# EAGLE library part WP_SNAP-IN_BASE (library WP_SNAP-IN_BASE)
SIERRA WIRELESS - WP SNAP-IN BASE - SNAP-IN SOCKET BASE FOR WP SERIES MCU Source: Datasheet
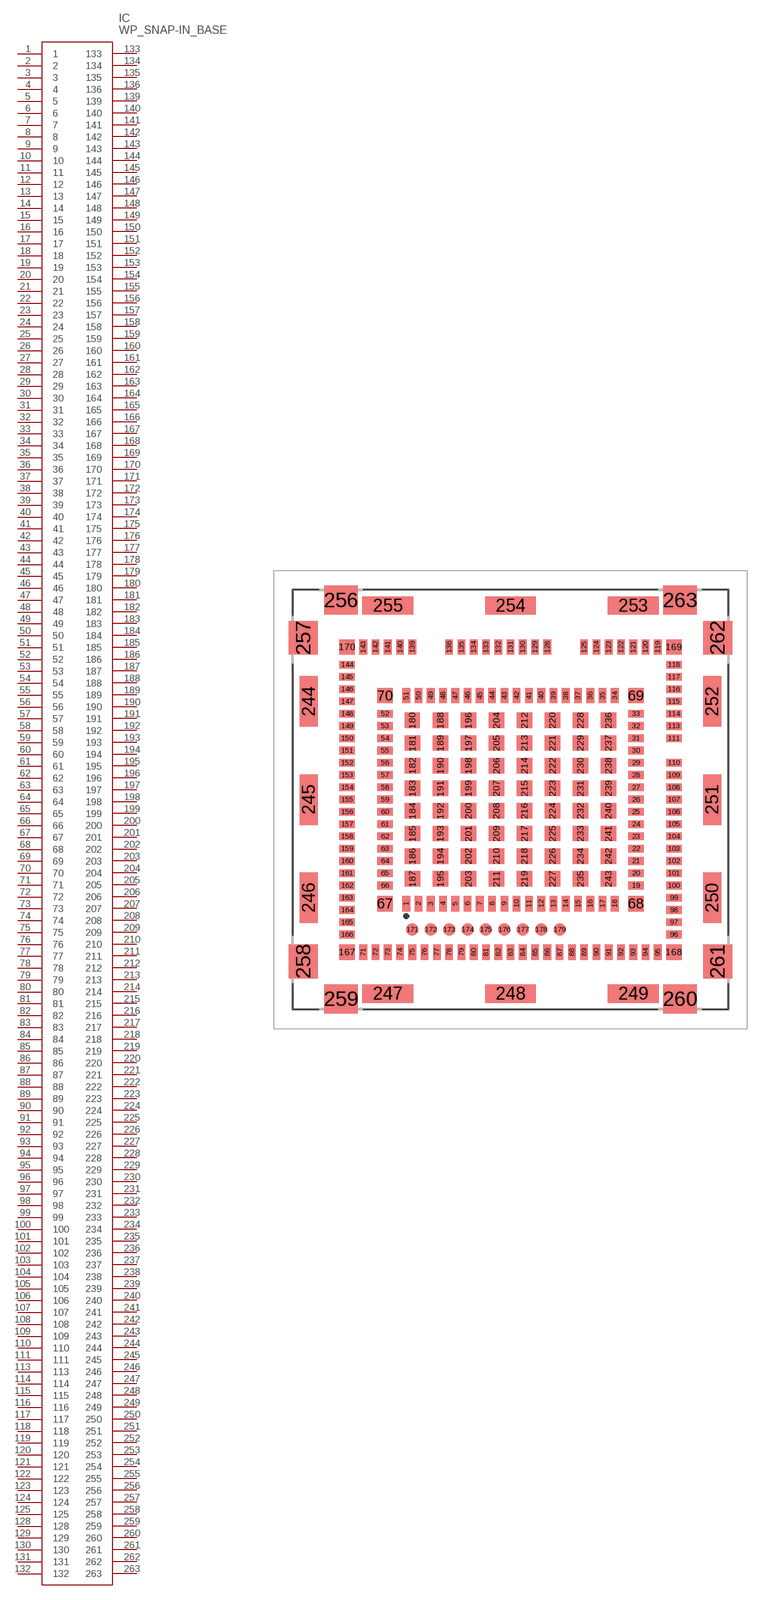
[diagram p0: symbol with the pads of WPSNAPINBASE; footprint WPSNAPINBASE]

Designator prefix IC

## WP_SNAP-IN_BASE (Arrow_Part_Number: WP SNAP-IN BASE; Description: SIERRA WIRELESS - WP SNAP-IN BASE - SNAP-IN SOCKET BASE FOR WP SERIES MCU; Height: 4mm; Manufacturer_Name: SIERRA WIRELESS; Manufacturer_Part_Number: WP SNAP-IN BASE)  [WPSNAPINBASE]
1  1
2  2
3  3
4  4
5  5
6  6
7  7
8  8
9  9
10  10
11  11
12  12
13  13
14  14
15  15
16  16
17  17
18  18
19  19
20  20
21  21
22  22
23  23
24  24
25  25
26  26
27  27
28  28
29  29
30  30
31  31
32  32
33  33
34  34
35  35
36  36
37  37
38  38
39  39
40  40
41  41
42  42
43  43
44  44
45  45
46  46
47  47
48  48
49  49
50  50
51  51
52  52
53  53
54  54
55  55
56  56
57  57
58  58
59  59
60  60
61  61
62  62
63  63
64  64
65  65
66  66
67  67
68  68
69  69
70  70
71  71
72  72
73  73
74  74
75  75
76  76
77  77
78  78
79  79
80  80
81  81
82  82
83  83
84  84
85  85
86  86
87  87
88  88
89  89
90  90
91  91
92  92
93  93
94  94
95  95
96  96
97  97
98  98
99  99
100  100
101  101
102  102
103  103
104  104
105  105
106  106
107  107
108  108
109  109
110  110
111  111
113  113
114  114
115  115
116  116
117  117
118  118
119  119
120  120
121  121
122  122
123  123
124  124
125  125
128  128
129  129
130  130
131  131
132  132
133  133
134  134
135  135
136  136
139  139
140  140
141  141
142  142
143  143
144  144
145  145
146  146
147  147
148  148
149  149
150  150
151  151
152  152
153  153
154  154
155  155
156  156
157  157
158  158
159  159
160  160
161  161
162  162
163  163
164  164
165  165
166  166
167  167
168  168
169  169
170  170
171  171
172  172
173  173
174  174
175  175
176  176
177  177
178  178
179  179
180  180
181  181
182  182
183  183
184  184
185  185
186  186
187  187
188  188
189  189
190  190
191  191
192  192
193  193
194  194
195  195
196  196
197  197
198  198
199  199
200  200
201  201
202  202
203  203
204  204
205  205
206  206
207  207
208  208
209  209
210  210
211  211
212  212
213  213
214  214
215  215
216  216
217  217
218  218
219  219
220  220
221  221
222  222
223  223
224  224
225  225
226  226
227  227
228  228
229  229
230  230
231  231
232  232
233  233
234  234
235  235
236  236
237  237
238  238
239  239
240  240
241  241
242  242
243  243
244  244
245  245
246  246
247  247
248  248
249  249
250  250
251  251
252  252
253  253
254  254
255  255
256  256
257  257
258  258
259  259
260  260
261  261
262  262
263  263

## Footprint WPSNAPINBASE (pad centres in mm)
WP SNAP-IN BASE
smd 0.5 x 1: 1 -6.8,-6.78; 2 -6,-6.78; 3 -5.2,-6.78; 4 -4.4,-6.78; 5 -3.6,-6.78; 6 -2.8,-6.78; 7 -2,-6.78; 8 -1.2,-6.78; 9 -0.4,-6.78; 10 0.4,-6.78; 11 1.2,-6.78; 12 2,-6.78; 13 2.8,-6.78; 14 3.6,-6.78; 15 4.4,-6.78; 16 5.2,-6.78; 17 6,-6.78; 18 6.8,-6.78; 34 6.8,6.78; 35 6,6.78; 36 5.2,6.78; 37 4.4,6.78; 38 3.6,6.78; 39 2.8,6.78; 40 2,6.78; 41 1.2,6.78; 42 0.4,6.78; 43 -0.4,6.78; 44 -1.2,6.78; 45 -2,6.78; 46 -2.8,6.78; 47 -3.6,6.78; 48 -4.4,6.78; 49 -5.2,6.78; 50 -6,6.78; 51 -6.8,6.78; 71 -9.6,-9.95; 72 -8.8,-9.95; 73 -8,-9.95; 74 -7.2,-9.95; 75 -6.4,-9.95; 76 -5.6,-9.95; 77 -4.8,-9.95; 78 -4,-9.95; 79 -3.2,-9.95; 80 -2.4,-9.95; 81 -1.6,-9.95; 82 -0.8,-9.95; 83 0,-9.95; 84 0.8,-9.95; 85 1.6,-9.95; 86 2.4,-9.95; 87 3.2,-9.95; 88 4,-9.95; 89 4.8,-9.95; 90 5.6,-9.95; 91 6.4,-9.95; 92 7.2,-9.95; 93 8,-9.95; 94 8.8,-9.95; 95 9.6,-9.95; 119 9.6,9.95; 120 8.8,9.95; 121 8,9.95; 122 7.2,9.95; 123 6.4,9.95; 124 5.6,9.95; 125 4.8,9.95; 128 2.4,9.95; 129 1.6,9.95; 130 0.8,9.95; 131 0,9.95; 132 -0.8,9.95; 133 -1.6,9.95; 134 -2.4,9.95; 135 -3.2,9.95; 136 -4,9.95; 139 -6.4,9.95; 140 -7.2,9.95; 141 -8,9.95; 142 -8.8,9.95; 143 -9.6,9.95
smd 1 x 0.5: 19 8.18,-5.6; 20 8.18,-4.8; 21 8.18,-4; 22 8.18,-3.2; 23 8.18,-2.4; 24 8.18,-1.6; 25 8.18,-0.8; 26 8.18,0; 27 8.18,0.8; 28 8.18,1.6; 29 8.18,2.4; 30 8.18,3.2; 31 8.18,4; 32 8.18,4.8; 33 8.18,5.6; 52 -8.18,5.6; 53 -8.18,4.8; 54 -8.18,4; 55 -8.18,3.2; 56 -8.18,2.4; 57 -8.18,1.6; 58 -8.18,0.8; 59 -8.18,0; 60 -8.18,-0.8; 61 -8.18,-1.6; 62 -8.18,-2.4; 63 -8.18,-3.2; 64 -8.18,-4; 65 -8.18,-4.8; 66 -8.18,-5.6; 96 10.65,-8.8; 97 10.65,-8; 98 10.65,-7.2; 99 10.65,-6.4; 100 10.65,-5.6; 101 10.65,-4.8; 102 10.65,-4; 103 10.65,-3.2; 104 10.65,-2.4; 105 10.65,-1.6; 106 10.65,-0.8; 107 10.65,0; 108 10.65,0.8; 109 10.65,1.6; 110 10.65,2.4; 111 10.65,4; 113 10.65,4.8; 114 10.65,5.6; 115 10.65,6.4; 116 10.65,7.2; 117 10.65,8; 118 10.65,8.8; 144 -10.65,8.8; 145 -10.65,8; 146 -10.65,7.2; 147 -10.65,6.4; 148 -10.65,5.6; 149 -10.65,4.8; 150 -10.65,4; 151 -10.65,3.2; 152 -10.65,2.4; 153 -10.65,1.6; 154 -10.65,0.8; 155 -10.65,0; 156 -10.65,-0.8; 157 -10.65,-1.6; 158 -10.65,-2.4; 159 -10.65,-3.2; 160 -10.65,-4; 161 -10.65,-4.8; 162 -10.65,-5.6; 163 -10.65,-6.4; 164 -10.65,-7.2; 165 -10.65,-8; 166 -10.65,-8.8
smd 1 x 1: 67 -8.18,-6.78; 68 8.18,-6.78; 69 8.18,6.78; 70 -8.18,6.78; 167 -10.65,-9.95; 168 10.65,-9.95; 169 10.65,9.95; 170 -10.65,9.95; 180 -6.4,5.162; 181 -6.388,3.688; 182 -6.388,2.213; 183 -6.388,0.737; 184 -6.388,-0.737; 185 -6.388,-2.213; 186 -6.388,-3.688; 187 -6.388,-5.163; 188 -4.563,5.162; 189 -4.563,3.688; 190 -4.563,2.213; 191 -4.563,0.737; 192 -4.563,-0.737; 193 -4.563,-2.213; 194 -4.563,-3.688; 195 -4.563,-5.163; 196 -2.738,5.162; 197 -2.738,3.688; 198 -2.738,2.213; 199 -2.738,0.737; 200 -2.738,-0.737; 201 -2.738,-2.213; 202 -2.738,-3.688; 203 -2.738,-5.163; 204 -0.913,5.162; 205 -0.913,3.688; 206 -0.913,2.213; 207 -0.913,0.737; 208 -0.913,-0.737; 209 -0.913,-2.213; 210 -0.913,-3.688; 211 -0.913,-5.163; 212 0.912,5.162; 213 0.912,3.688; 214 0.912,2.213; 215 0.912,0.737; 216 0.912,-0.737; 217 0.912,-2.213; 218 0.912,-3.688; 219 0.912,-5.163; 220 2.737,5.162; 221 2.737,3.688; 222 2.737,2.213; 223 2.737,0.737; 224 2.737,-0.737; 225 2.737,-2.213; 226 2.737,-3.688; 227 2.737,-5.163; 228 4.562,5.162; 229 4.562,3.688; 230 4.562,2.213; 231 4.562,0.737; 232 4.562,-0.737; 233 4.562,-2.213; 234 4.562,-3.688; 235 4.562,-5.163; 236 6.388,5.162; 237 6.388,3.688; 238 6.388,2.213; 239 6.388,0.737; 240 6.388,-0.737; 241 6.388,-2.213; 242 6.388,-3.688; 243 6.388,-5.163
smd 0.8 x 0.8: 171 -6.4,-8.48; 172 -5.2,-8.48; 173 -4,-8.48; 174 -2.8,-8.48; 175 -1.6,-8.48; 176 -0.4,-8.48; 177 0.8,-8.48; 178 2,-8.48; 179 3.2,-8.48
smd 1.2 x 3.3: 244 -13.15,6.4; 245 -13.15,0; 246 -13.15,-6.4; 250 13.15,-6.4; 251 13.15,0; 252 13.15,6.4
smd 3.3 x 1.2: 247 -8,-12.65; 248 0,-12.65; 249 8,-12.65; 253 8,12.65; 254 0,12.65; 255 -8,12.65
smd 2.2 x 1.9: 256 -11.05,13; 259 -11.05,-13; 260 11.05,-13; 263 11.05,13
smd 1.9 x 2.2: 257 -13.5,10.55; 258 -13.5,-10.55; 261 13.5,-10.55; 262 13.5,10.55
